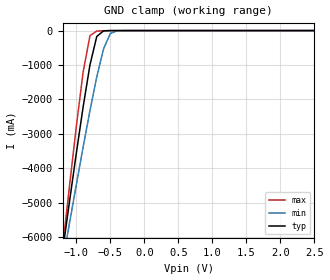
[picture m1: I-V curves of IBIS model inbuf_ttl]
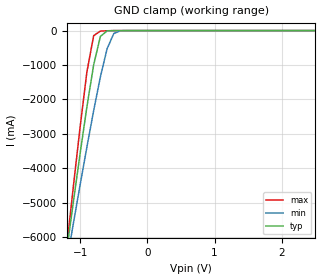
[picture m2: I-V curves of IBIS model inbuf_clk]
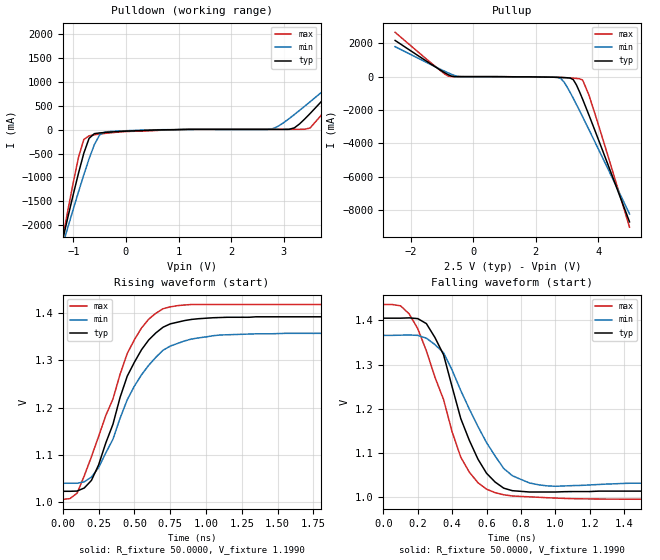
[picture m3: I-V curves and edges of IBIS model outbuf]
| IBIS file 5t9310z.ibs created by s2ibis2 version 1.2
| North Carolina State University Electronics Research Laboratory  1995
[IBIS ver]   2.1
[File name]   5t9310z.ibs
[File Rev]   1.1
[Date]   10/05/2004 smg
[Source]   Integrated Device Technology, Inc.
[Notes]   1.Temperatures: typ=25C, min=125C, max=-40C 2.RRmp rates based
   on 100 ohm load.
[Disclaimer] Integrated Device Technology, Inc. ("IDT") hereby grants the
   user of this IBIS model a non-exclusive, nontransferable
   license to use this IBIS model under the following terms. The
   user is granted this license only to use the IBIS model and is
   not granted rights to sell, copy (except as needed to run the
   IBIS model), rent, lease or sub-license the IBIS model in
   whole or in part, or in modified form to anyone. The User may
   modify the IBIS model to suit its specific applications, but
   rights to derivative works and such modifications shall belong
   to IDT. This IBIS model is provided on an AS IS" basis and IDT
   makes absolutely no warranty with respect to the information
   contained herein. IDT DISCLAIMS AND CUSTOMER WAIVES ALL
   WARRANTIES, EXPRESS AND IMPLIED, INCLUDING WARRANTIES OF
   MERCHANTABILITY AND FITNESS FOR A PARTICULAR PURPOSE. THE
   ENTIRE RISK AS TO QUALITY AND PERFORMANCE IS WITH THE USER
   ACCORDINGLY, IN NO EVENT SHALL IDT BE LIABLE FOR ANY DIRECT OR
   INDIRECT DAMAGES, WHETHER IN CONTRACT OR TORT, INCLUDING ANY
   LOST PROFITS OR OTHER INCIDENTAL, CONSEQUENTIAL, EXEMPLARY, OR
   PUNITIVE DAMAGES ARISING OUT OF THE USE OR APPLICATION OF THE
   IBIS model. Further, IDT reserves the right to make changes
   without notice to any product herein to improve reliability,
   function, or design. IDT does not convey any license under
   patent rights or any other intellectual property rights,
   including those of third parties. IDT is not obligated to
   provide maintenance or support for the licensed IBIS model.
[Copyright]   Copyright 1997, Integrated Device Technology, Inc. all rights
   reserved
|   Component IDT5T9310Z
[Component]   idt5t9310z
[Manufacturer]   Integrated Device Technology, Inc.
[Package]
| variable   typ   min   max
R_pkg   86.0000m   61.00000m   0.11300
L_pkg   2.10000nH   1.50000nH   2.70000nH
C_pkg   0.20000pF   0.16000pF   0.24000pF
[Pin]  signal_name   model_name   R_pin   L_pin   C_pin
0   GND   GND
1   G1X   inbuf_ttl
2   VDD   POWER
3   GND   GND
4   Q1   outbuf
5   Q1X   outbuf
6   Q2   outbuf
7   Q2X   outbuf
8   VDD   POWER
9   A1   inbuf_clk
10   A1X   inbuf_clk
11   GL   inbuf_ttl
12   VDD   POWER
13   Q3   outbuf
14   Q3X   outbuf
15   Q4   outbuf
16   Q5X   outbuf
17   Q5   outbuf
18   Q5X   outbuf
19   VDD   POWER
20   GND   GND
21   A2X   inbuf_clk
22   A2   inbuf_clk
23   VDD   POWER
24   Q6X   outbuf
25   Q6   outbuf
26   Q7X   outbuf
27   Q7   outbuf
28   VDD   POWER
29   PDX   inbuf_ttl
30   G2X   inbuf_ttl
31   GND   GND
32   VDD   POWER
33   Q8X   outbuf
34   Q8   outbuf
35   Q9X   outbuf
36   Q9   outbuf
37   Q10X   outbuf
38   Q10   outbuf
39   VDD   POWER
40   SEL   inbuf_ttl
[Diff Pin]  inv_pin  vdiff   tdelay_typ  tdelay_min  tdelay_max
  4   5   0mV   NA   NA   NA  | Output pair
  6   7   0mV   NA   NA   NA  | Output pair
  9   10   100mV   NA   NA   NA  | Input  pair
 13   14   0mV   NA   NA   NA  | Output pair
 15   16   0mV   NA   NA   NA  | Output pair
 17   18   0mV   NA   NA   NA  | Output pair
 22   21   100mV   NA   NA   NA  | Input  pair
 25   24   0mV   NA   NA   NA  | Output pair
 34   33   0mV   NA   NA   NA  | Output pair
 36   35   0mV   NA   NA   NA  | Output pair
 38   37   0mV   NA   NA   NA  | Output pair
| Models and submodels in the file (3): inbuf_ttl (Input), inbuf_clk (Input), outbuf (Output)
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|   Model inbuf_ttl
[Model]   inbuf_ttl
Model_type   Input
Polarity   Non-Inverting
Vinl =   0.7000V
Vinh =   1.7000V
C_comp   3.0000pF   NA   NA
[Temperature Range]   25.0000   0.1250k   -40.0000
[Voltage Range]   2.5000V   2.3000V   2.7000V
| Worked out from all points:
|   GND clamp passes 1 mA (typ) near -0.50 V on its own axis
[GND_clamp]
| voltage   I(typ)   I(min)   I(max)
-2.5V     -25.73A    -21.91A    -30.44A
-1.2V     -6.384A    -6.715A    -6.273A
-1.1V     -4.953A    -5.584A    -4.495A
-1V       -3.554A    -4.47A     -2.775A
-900mV    -2.21A     -3.379A    -1.196A
-800mV    -995.8mA   -2.327A    -147.4mA
-700mV    -170.9mA   -1.346A    -14.56mA
-600mV    -7.9mA     -528mA     -5.356mA
-500mV    -649.8uA   -83.93mA   -1.004mA
-400mV    -51.46uA   -5.547mA   -73.83uA
2.5V      109pA      123nA      9.328pA
[POWER_clamp]
| voltage   I(typ)   I(min)   I(max)
-2.5V     0A         0A         0A
-2.4V     0A         0A         0A
-2.3V     0A         0A         0A
0V        0A         0A         0A
|   Model inbuf_clk
[Model]   inbuf_clk
Model_type   Input
Polarity   Non-Inverting
Vinl =  0.000V
Vinh =   2.5000V
C_comp   3.0000pF   NA   NA
[Temperature Range]   25.0000   0.1250k   -40.0000
[Voltage Range]   2.5000V   2.3000V   2.7000V
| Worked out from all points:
|   GND clamp passes 1 mA (typ) near -0.50 V on its own axis
[GND_clamp]
| voltage   I(typ)   I(min)   I(max)
-2.5V     -25.73A    -21.91A    -30.45A
-1.2V     -6.384A    -6.715A    -6.273A
-1.1V     -4.953A    -5.585A    -4.495A
-1V       -3.554A    -4.47A     -2.775A
-900mV    -2.211A    -3.379A    -1.196A
-800mV    -996mA     -2.327A    -147.5mA
-700mV    -171mA     -1.346A    -14.62mA
-600mV    -7.914mA   -528.1mA   -5.379mA
-500mV    -651uA     -83.95mA   -1.007mA
-400mV    -51.48uA   -5.549mA   -73.85uA
2.5V      109pA      123nA      9.327pA
[POWER_clamp]
| voltage   I(typ)   I(min)   I(max)
-2.5V     0A         0A         0A
-2.4V     0A         0A         0A
-2.3V     0A         0A         0A
0V        0A         0A         0A
|   Model outbuf
[Model]   outbuf
Model_type   Output
Polarity   Non-Inverting
Vmeas =   1.2000V
Rref =  50.0000
C_comp   3.0000pF   NA   NA
[Temperature Range]   25.0000   0.1250k   -40.0000
[Voltage Range]   2.5000V   2.3000V   2.7000V
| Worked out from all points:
|   slope of the pulldown table from 0 to 0.375 V, typ, clamps not added: 24.4 ohm
|   slope of the pullup table from 0 to 0.375 V, typ, clamps not added: 877 ohm
|   rising waveform, R_fixture 50.0000, V_fixture 1.1990: 20-80 % time 272ps typ, 313ps min, 296ps max; typ from 1.02 V to 1.39 V
|   falling waveform, R_fixture 50.0000, V_fixture 1.1990: 20-80 % time 198ps typ, 254ps min, 227ps max; typ from 1.41 V to 1.01 V
[Pulldown]
| voltage   I(typ)   I(min)   I(max)
-2.5V     -8.706A    -7.447A    -10.26A
-1.3V     -2.775A    -2.787A    -2.859A
-1.1V     -1.819A    -2.032A    -1.671A
-900mV    -904.7mA   -1.297A    -573mA
-800mV    -491.1mA   -943.2mA   -203.9mA
-700mV    -180.1mA   -608.1mA   -127.2mA
-400mV    -57.62mA   -46.81mA   -76.96mA
2.7V      7.511mA    8.286mA    8.594mA
3.2V      38.72mA    317.7mA    8.189mA
3.5V      339.8mA    586.3mA    36.21mA
4.9V      2.045A     1.896A     2.176A
5V        2.17A      1.99A      2.337A
[Pullup]
| voltage   I(typ)   I(min)   I(max)
-2.5V     2.172A     1.801A     2.659A
-800mV    118.3mA    227.8mA    33.19mA
-400mV    2.286mA    3.233mA    3.84mA
2.7V      -40.07mA   -44.52mA   -38mA
2.8V      -47.2mA    -107.7mA   -44.88mA
2.9V      -55.09mA   -310.9mA   -53.76mA
3.2V      -177.8mA   -1.296A    -87.74mA
3.3V      -490mA     -1.66A     -104mA
3.5V      -1.353A    -2.407A    -201.8mA
3.7V      -2.294A    -3.168A    -1.099A
3.9V      -3.26A     -3.937A    -2.259A
5V        -8.703A    -8.23A     -9.019A
[Ramp]
| variable   typ   min   max
dV/dt_r   0.2214/0.2553n   0.1902/0.2997n   0.2472/0.2817n
dV/dt_f   0.2346/0.1939n   0.1998/0.2485n   0.2650/0.2125n
R_load = 50.0000
[Rising Waveform]
R_fixture = 50.0000
V_fixture = 1.1990
| time   V(typ)   V(min)   V(max)
0s        1.023V     1.04V      1.006V
100ps     1.024V     1.04V      1.019V
200ps     1.046V     1.053V     1.096V
350ps     1.165V     1.133V     1.218V
450ps     1.266V     1.216V     1.315V
550ps     1.323V     1.27V      1.369V
700ps     1.37V      1.321V     1.409V
850ps     1.384V     1.341V     1.417V
1.1ns     1.391V     1.353V     1.418V
2.5ns     1.392V     1.357V     1.418V
[Falling Waveform]
R_fixture = 50.0000
V_fixture = 1.1990
| time   V(typ)   V(min)   V(max)
0s        1.405V     1.366V     1.436V
100ps     1.405V     1.367V     1.433V
150ps     1.406V     1.367V     1.415V
250ps     1.393V     1.36V      1.331V
350ps     1.322V     1.327V     1.22V
450ps     1.177V     1.241V     1.09V
600ps     1.054V     1.123V     1.018V
750ps     1.014V     1.048V     1.002V
950ps     1.011V     1.025V     998.1mV
2.5ns     1.014V     1.033V     994.4mV
